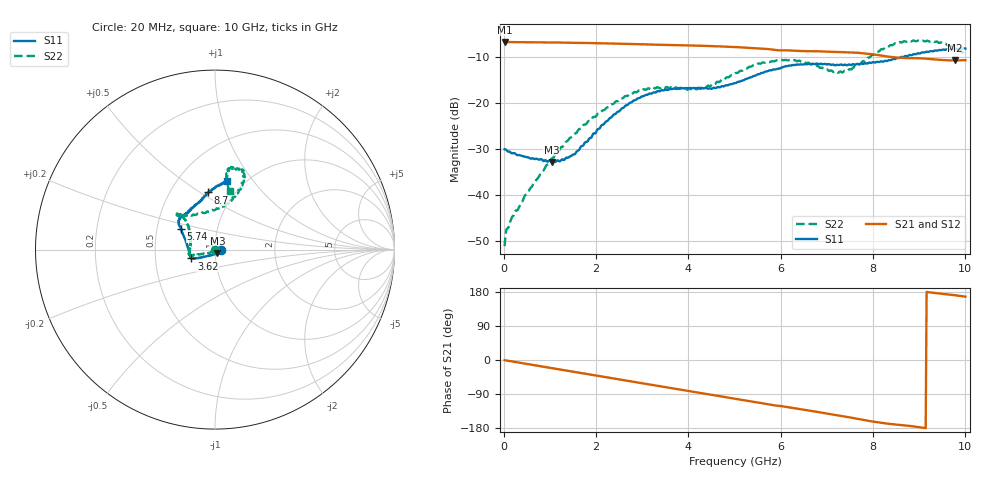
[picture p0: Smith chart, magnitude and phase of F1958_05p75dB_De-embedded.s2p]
! Integrated Device Technology
! Corporate Headquarters
! 6024 Silver Creek Valley Road
! San Jose, CA 95138  USA
! Phone:  1-408-284-8200
! Toll Free:  1-800-223-1366
! Webpage:  http://www.idt.com/
! Timing and RF Division
! 515 Groton Road, Suite 102
! Westford, MA 01886-6024
! Device:  F1958
! Description: 7-bit 0.25 dB Digital Step Attenuator
! Frequency:  0.001 -  6.000 GHz
! Package:  4x4 mm Thin QFN Plastic Package: 24 pin
! Ports:  2 RF, 12 DC
!  Pin  1  = D0
!  Pin  2  = VDD
!  Pin  3  = VMODE
!  Pin  4  = GND
!  Pin  5  = RF1  =  Port 1
!  Pin  6  = GND
!  Pin  7  = GND
!  Pin  8  = GND
!  Pin  9  = GND
!  Pin 10  = GND
!  Pin 11  = GND
!  Pin 12  = GND
!  Pin 13  = GND
!  Pin 14  = RF2  =  Port 2
!  Pin 15  = GND
!  Pin 16  = LE
!  Pin 17  = CLK
!  Pin 18  = DATA
!  Pin 19  = D6
!  Pin 20  = D5
!  Pin 21  = D4
!  Pin 22  = D3
!  Pin 23  = D2
!  Pin 24  = D1
! State:  23
! Atten State:  5.75 dB
! Voltage:  +3.30 Volts
! Current:  0.258 mA
! Data:  The device was measured on a F1958 evaluation board which has
!  individual transmission lines to the RF pins.  Data was collected
!  using a calibrated network analyzer.  The evaluation board was
!  de-embedded using Automatic Fixture Removal (AFR).
!  The reference plane is the edge of the package pin.
! Misc:
!  Action Tracker AT0419
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# GHz S dB R 50
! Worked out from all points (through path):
!   500 points, 20 MHz to 10 GHz, reference 50 ohm
!   highest |S21| = -6.83 dB at 20 MHz (marker M1); lowest = -10.9 dB at 9.78 GHz (marker M2)
!   group delay of S21, straight-line fit = 54.7 ps
!   lowest |S11| = -32.9 dB at 1.04 GHz (marker M3), VSWR 1.05, Z = 51.3 - j1.9 ohm
!   |S11| at or under -10 dB: start of sweep to 8.677 GHz
!   |S22| runs from -51.2 to -6.5 dB; largest |S21 - S12| = 0.0012
!   S11 on the Smith chart (normalised r, x): 20 MHz: 1.06, -0.00; 3.62 GHz: 0.76, -0.08; 5.74 GHz: 0.67, +0.16; 8.7 GHz: 0.76, +0.54; 10 GHz: 0.84, +0.75
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0.02  -30.14 -3.8  -6.83 -0.6  -6.83 -0.5  -51.20 -140.2
0.08  -30.55 -6.1  -6.85 -1.8  -6.85 -1.8  -47.35 -130.1
0.22  -30.97 -10.7  -6.87 -4.7  -6.87 -4.7  -44.47 -136.7
1.04  -32.93 -55.0  -6.94 -21.4  -6.94 -21.4  -32.12 -143.0
1.42  -31.82 -94.4  -7.00 -29.2  -6.99 -29.2  -27.83 -152.0
1.7  -29.42 -115.9  -7.04 -34.8  -7.04 -34.8  -25.33 -157.5
2.6  -21.07 -150.0  -7.24 -53.2  -7.22 -53.2  -18.88 -165.5
3.36  -17.54 -157.8  -7.44 -68.7  -7.44 -68.8  -16.81 -168.4
3.62  -17.06 -159.3  -7.50 -73.9  -7.50 -74.0  -16.64 -174.4
4.3  -16.81 -169.9  -7.66 -87.7  -7.68 -87.7  -16.80 160.4
5.02  -15.77 167.0  -7.94 -102.4  -7.95 -102.4  -13.58 137.6
5.74  -13.07 148.5  -8.39 -117.1  -8.40 -117.1  -11.16 135.3
6.28  -11.83 142.8  -8.73 -127.0  -8.75 -126.9  -10.81 136.9
6.68  -11.57 137.8  -8.85 -134.5  -8.86 -134.4  -11.68 132.5
7.1  -11.80 131.2  -8.98 -143.5  -8.99 -143.4  -13.04 115.6
7.38  -11.77 127.2  -9.06 -149.0  -9.07 -148.9  -13.08 94.5
7.9  -11.39 115.1  -9.39 -160.4  -9.39 -160.4  -10.25 71.4
8.34  -10.78 104.8  -10.03 -168.4  -10.03 -168.5  -7.82 67.0
8.7  -9.87 97.1  -10.34 -172.7  -10.33 -172.7  -6.72 70.9
9.3  -8.85 85.3  -10.58 177.3  -10.59 177.3  -6.69 80.2
9.78  -8.28 81.0  -10.86 170.8  -10.88 170.8  -8.10 80.0
10  -8.27 79.9  -10.78 167.2  -10.81 167.3  -9.49 75.6
